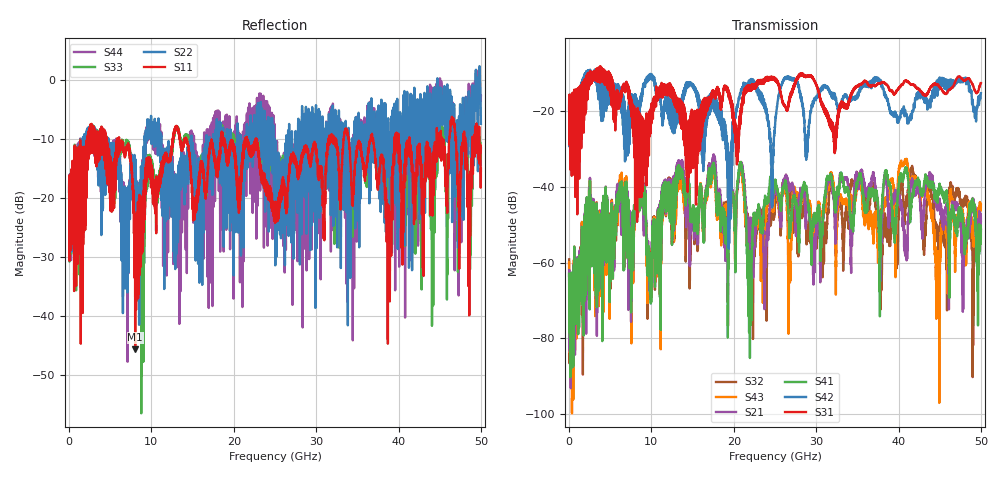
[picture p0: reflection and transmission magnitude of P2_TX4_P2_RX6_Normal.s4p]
!Keysight Technologies,N5225B,MY57041031,A.13.20.10
!Date: Friday, May 31, 2019 11:36:07
!Correction: S11(Full 4 Port(1,2,3,4))
!S12(Full 4 Port(1,2,3,4))
!S13(Full 4 Port(1,2,3,4))
!S14(Full 4 Port(1,2,3,4))
!S21(Full 4 Port(1,2,3,4))
!S22(Full 4 Port(1,2,3,4))
!S23(Full 4 Port(1,2,3,4))
!S24(Full 4 Port(1,2,3,4))
!S31(Full 4 Port(1,2,3,4))
!S32(Full 4 Port(1,2,3,4))
!S33(Full 4 Port(1,2,3,4))
!S34(Full 4 Port(1,2,3,4))
!S41(Full 4 Port(1,2,3,4))
!S42(Full 4 Port(1,2,3,4))
!S43(Full 4 Port(1,2,3,4))
!S44(Full 4 Port(1,2,3,4))
!S4P File: Measurements: <S11,S12,S13,S14>,
!<S21,S22,S23,S24>,
!<S31,S32,S33,S34>,
!<S41,S42,S43,S44>:
# Hz S  dB  R 50.0
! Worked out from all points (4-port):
!   5000 points, 10 MHz to 50 GHz, reference 50 ohm
!   strongest paths, dB at 10 MHz, 12.51 GHz, 25.01 GHz, 37.51 GHz, 50 GHz:
!     S31: -19.4, -14.3, -11.3, -12.8, -12.5
!     S42: -19.5, -16.8, -23.8, -11.5, -15.2
!     S41: -62.9, -45.6, -38.3, -45.1, -51.4
!     S21: -63.6, -43.9, -40.7, -44.1, -49.1
!     S43: -60.0, -45.8, -39.1, -60.0, -44.7
!     S32: -59.1, -44.2, -44.0, -49.2, -51.0
!   lowest |S11| = -45.6 dB at 8.03 GHz (marker M1), VSWR 1.01, Z = 50.2 - j0.474 ohm
!   |S11| at or under -10 dB: 6.073 GHz to 12.61 GHz (6.542 GHz wide, 70 % of centre); 14.21 GHz to 18.43 GHz (4.228 GHz wide, 25.9 % of centre); 22.71 GHz to 31.52 GHz (8.805 GHz wide, 32.5 % of centre)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
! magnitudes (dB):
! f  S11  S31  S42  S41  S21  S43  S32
! 10 MHz  -18.9  -19.4  -19.5  -62.9  -63.6  -60.0  -59.1
! 8.03 GHz  -45.6  -23.4  -18.6  -45.2  -45.4  -46.1  -46.5
! 20.86 GHz  -17.8  -19.1  -14.8  -33.5  -33.6  -34.5  -34.4
! 21.93 GHz  -11.6  -14.6  -12.6  -58.6  -52.3  -56.1  -52.5
! 40.84 GHz  -12.4  -11.9  -20.6  -35.3  -55.3  -32.8  -46.4
! 44.77 GHz  -9.7  -13.1  -13.0  -42.6  -45.0  -57.8  -52.5
! 50 GHz  -15.1  -12.5  -15.2  -51.4  -49.1  -44.7  -51.0
